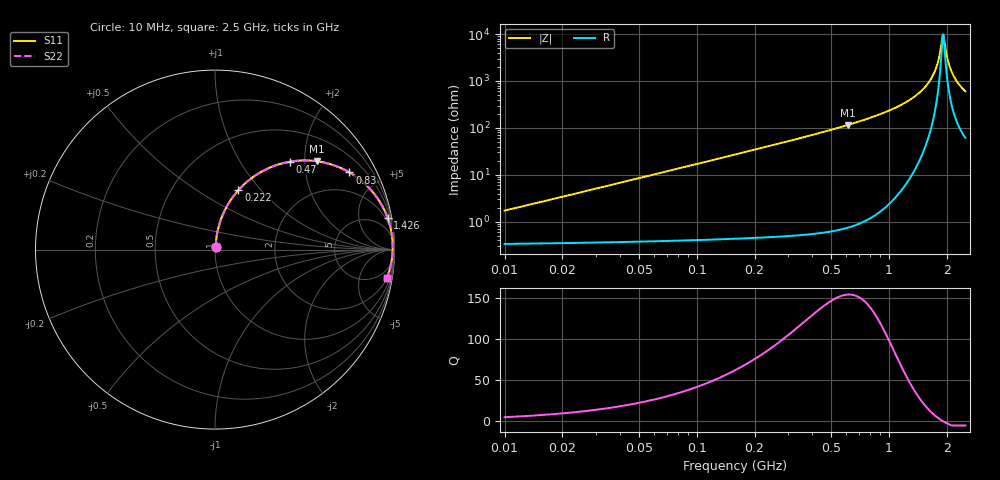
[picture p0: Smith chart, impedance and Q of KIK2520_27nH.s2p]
!version-2
!date-01.2022
!Series
# MHz S RI R 50
!Freq ReS11 ImS11 ReS21 ImS21 ReS12 ImS12 ReS22 ImS22
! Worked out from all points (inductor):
!   624 points, 10 MHz to 2.5 GHz, reference 50 ohm
!   read as one part in series: L = 27 nH near 22 MHz
!   highest Q = 154 at 610 MHz (marker M1), where L = 30.1 nH
!   self-resonance near 1.914 GHz
!   S11 on the Smith chart (normalised r, x): 10 MHz: 1.01, +0.03; 222 MHz: 1.01, +0.76; 470 MHz: 1.01, +1.70; 830 MHz: 1.03, +3.47; 1.426 GHz: 1, +11; 2.5 GHz: 2, -12
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10  0.00365 0.0168  0.9964 -0.0168  0.9964 -0.0168  0.00365 0.0168
38  0.00776 0.0638  0.9922 -0.0638  0.9922 -0.0638  0.00776 0.0638
74  0.0193 0.1228  0.9807 -0.1228  0.9807 -0.1228  0.0193 0.1228
134  0.0532 0.2154  0.9468 -0.2154  0.9468 -0.2154  0.0532 0.2154
222  0.1302 0.3305  0.8698 -0.3305  0.8698 -0.3305  0.1302 0.3305
426  0.3673 0.4784  0.6327 -0.4784  0.6327 -0.4784  0.3673 0.4784
470  0.4191 0.4899  0.5809 -0.4899  0.5809 -0.4899  0.4191 0.4899
610  0.5697 0.4919  0.4303 -0.4919  0.4303 -0.4919  0.5697 0.4919
830  0.7488 0.43  0.2512 -0.43  0.2512 -0.43  0.7488 0.43
842  0.7565 0.4254  0.2435 -0.4254  0.2435 -0.4254  0.7565 0.4254
1258  0.9295 0.2463  0.0705 -0.2463  0.0705 -0.2463  0.9295 0.2463
1426  0.9616 0.176  0.0384 -0.176  0.0384 -0.176  0.9616 0.176
1670  0.9851 0.0827  0.0149 -0.0827  0.0149 -0.0827  0.9851 0.0827
1802  0.9896 0.0369  0.0104 -0.0369  0.0104 -0.0369  0.9896 0.0369
1846  0.99 0.0223  0.00997 -0.0223  0.00997 -0.0223  0.99 0.0223
1898  0.99 0.00553  0.00999 -0.00553  0.00999 -0.00553  0.99 0.00553
1914  0.9899 0.00047  0.0101 -0.00047  0.0101 -0.00047  0.9899 0.00047
1930  0.9897 -0.00454  0.0103 0.00454  0.0103 0.00454  0.9897 -0.00454
2006  0.9882 -0.0277  0.0118 0.0277  0.0118 0.0277  0.9882 -0.0277
2086  0.9855 -0.0511  0.0145 0.0511  0.0145 0.0511  0.9855 -0.0511
2254  0.9767 -0.0968  0.0233 0.0968  0.0233 0.0968  0.9767 -0.0968
2500  0.9578 -0.1559  0.0422 0.1559  0.0422 0.1559  0.9578 -0.1559
